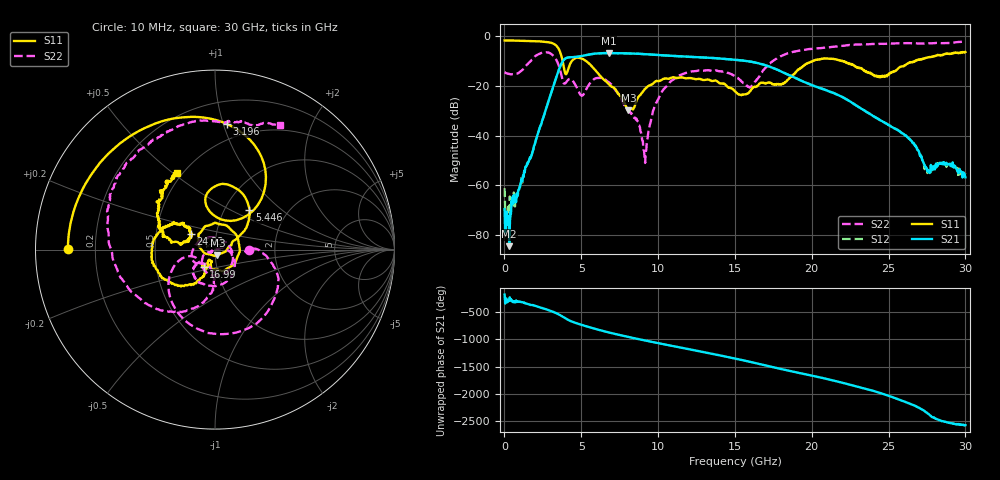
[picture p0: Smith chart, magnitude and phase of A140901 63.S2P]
!  2-Port S-parameters saved by WinCal
! VAR MeasName=S-Parameters (CALIBRATED_DATA) read from VNA (N5244A)
! VAR MeasDate=11/3/2014 9:37:01 AM
! VAR NAME=A140901 63
! VAR FILENAME=A140901 63.S2P
! VAR DATE=11/3/2014 9:37:01 AM
! VAR PHYS_PORTS=1,2
# Hz S RI R 50
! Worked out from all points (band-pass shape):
!   801 points, 10 MHz to 30 GHz, reference 50 ohm
!   highest |S21| = -6.78 dB at 6.795 GHz (marker M1); lowest = -84.5 dB at 309.9 MHz (marker M2)
!   |S21| within 3 dB of the highest: 3.831 GHz to 15.47 GHz (11.64 GHz wide, 121 % of centre)
!   lowest |S11| = -29.8 dB at 8.07 GHz (marker M3), VSWR 1.07, Z = 51.3 - j3.04 ohm
!   |S11| at or under -10 dB: 3.784 GHz to 4.385 GHz (601.3 MHz wide, 14.7 % of centre); 5.311 GHz to 20.06 GHz (14.75 GHz wide, 116 % of centre); 22 GHz to 26.73 GHz (4.726 GHz wide, 19.4 % of centre)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
!   |S22| runs from -51.0 to -2.1 dB; largest |S21 - S12| = 0.0019
!   S11 on the Smith chart (normalised r, x): 10 MHz: 0.10, +0.00; 3.196 GHz: 0.37, +1.03; 5.446 GHz: 1.30, +0.63; 16.99 GHz: 0.87, -0.17; 24.23 GHz: 0.75, +0.13; 30 GHz: 0.47, +0.52
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1e7  -0.819 0.00257  -0.000333 -2.11e-05  0.000406 -0.00078  0.1874 -0.00133
3.099e8  -0.8127 0.1008  1.12e-05 5.88e-05  0.000171 0.000209  0.1745 -0.0123
2.1093e9  -0.4914 0.6199  0.00786 -0.00504  0.0078 -0.00511  0.3438 -0.2337
3.196438e9  0.0649 0.7005  -0.0739 -0.0703  -0.0734 -0.0699  -0.22 -0.3319
3.6088e9  0.2839 0.4038  -0.2324 0.0532  -0.232 0.053  -0.2052 -0.0654
4.096138e9  -0.0122 0.1953  0.0297 0.3696  0.0294 0.3695  -0.1029 -0.0769
5.033325e9  0.1391 0.325  0.3867 -0.0977  0.3868 -0.0974  0.0186 0.0603
5.445688e9  0.192 0.2207  0.2773 -0.3205  0.2775 -0.3201  0.0976 -0.0207
6.795238e9  0.0985 0.0442  -0.4057 -0.2129  -0.4046 -0.2131  -0.0735 -0.0923
8.069812e9  0.0135 -0.0296  -0.257 0.3689  -0.258 0.3686  -0.0285 -0.014
9.15695e9  -0.0857 0.0133  0.2203 0.3741  0.2202 0.3741  -0.000611 0.00275
1.001916e10  -0.0847 0.0932  0.4117 0.0731  0.4112 0.0726  0.0539 0.00392
1.193102e10  0.1069 0.0952  -0.0375 -0.3841  -0.0378 -0.383  0.0708 -0.1729
1.343052e10  0.0842 -0.096  -0.3658 -0.00267  -0.3661 -0.00382  -0.0632 -0.1932
1.5005e10  -0.0394 -0.0668  0.00629 0.3347  0.00678 0.3341  -0.1181 -0.1026
1.597968e10  -0.0218 -0.0755  0.2713 0.1478  0.2716 0.1476  -0.0439 -0.0836
1.699184e10  -0.0623 -0.0958  0.2054 -0.1593  0.2054 -0.1592  -0.0149 -0.2293
2.002832e10  -0.255 -0.1785  -0.0704 0.0752  -0.0714 0.0748  -0.5421 -0.1181
2.422692e10  -0.1362 0.0852  -0.0216 -0.00663  -0.0217 -0.00656  -0.3793 0.5821
2.501416e10  -0.1611 0.0433  -0.00879 0.0137  -0.00886 0.0136  -0.2773 0.6518
2.763829e10  -0.3212 0.2003  -0.00152 0.00114  -0.0015 0.00107  0.0787 0.7132
3e10  -0.2098 0.4294  0.000856 -0.00117  0.000908 -0.00151  0.3613 0.6959
